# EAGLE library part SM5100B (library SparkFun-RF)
LinkSprite SM5100B GSM/GPRS Module The SM5100B is a miniature, quad-band GSM 850/EGSM 900/DCS 1800/PCS 1900 module, which can be integrated into a great number of wireless projects. You can use this module to accomplish almost anything a normal cell phone can - SMS text messages, GSM/GPRS, TCP/IP, and more! SparkFun Products GSM/GPRS Module - SM5100B (CEL-09533)
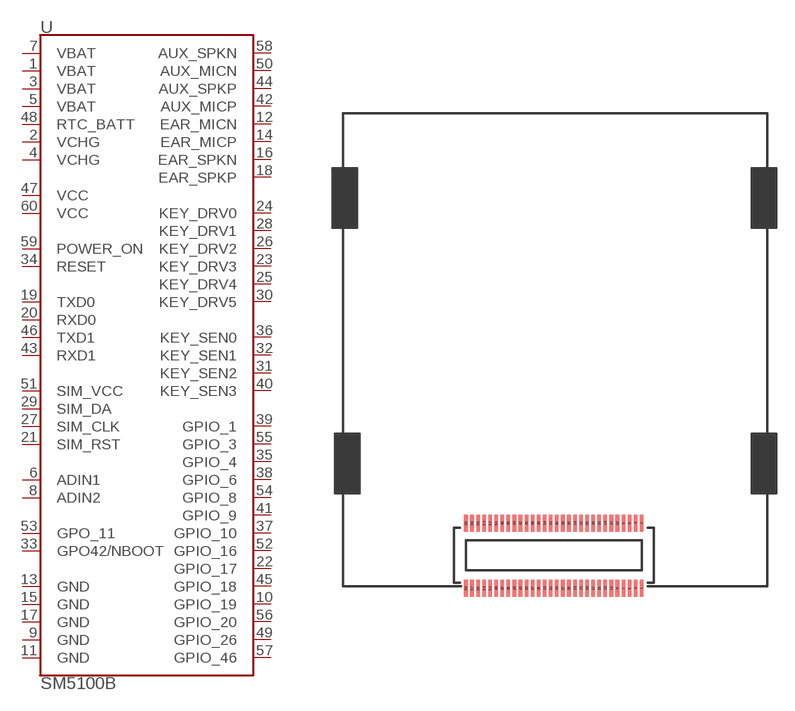
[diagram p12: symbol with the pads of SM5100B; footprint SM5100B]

Designator prefix -

## SM5100B (PROD_ID: CONN-09315)  [SM5100B]
1  VBAT
2  VCHG
3  VBAT
4  VCHG
5  VBAT
6  ADIN1
7  VBAT
8  ADIN2
9  GND
10  GPIO_19
11  GND
12  EAR_MICN
13  GND
14  EAR_MICP
15  GND
16  EAR_SPKN
17  GND
18  EAR_SPKP
19  TXD0
20  RXD0
21  SIM_RST
22  GPIO_17
23  KEY_DRV3
24  KEY_DRV0
25  KEY_DRV4
26  KEY_DRV2
27  SIM_CLK
28  KEY_DRV1
29  SIM_DA
30  KEY_DRV5
31  KEY_SEN2
32  KEY_SEN1
33  GPO42/NBOOT
34  RESET
35  GPIO_4
36  KEY_SEN0
37  GPIO_10
38  GPIO_6
39  GPIO_1
40  KEY_SEN3
41  GPIO_9
42  AUX_MICP
43  RXD1
44  AUX_SPKP
45  GPIO_18
46  TXD1
47  VCC
48  RTC_BATT
49  GPIO_26
50  AUX_MICN
51  SIM_VCC
52  GPIO_16
53  GPO_11
54  GPIO_8
55  GPIO_3
56  GPIO_20
57  GPIO_46
58  AUX_SPKN
59  POWER_ON
60  VCC

## Footprint SM5100B (pad centres in mm)
SM5100B GSM/GPRS Module - 60-pin 0.5mm-pitch board-to-board connector Mill layers define four shielding GND tabs. The SM5100B GSM/GPRS module interfaces with a board via a 60-pin board-to-board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
smd 0.3 x 1.4: 1 7.25,-2.68; 2 7.25,2.68; 3 6.75,-2.68; 4 6.75,2.68; 5 6.25,-2.68; 6 6.25,2.68; 7 5.75,-2.68; 8 5.75,2.68; 9 5.25,-2.68; 10 5.25,2.68; 11 4.75,-2.68; 12 4.75,2.68; 13 4.25,-2.68; 14 4.25,2.68; 15 3.75,-2.68; 16 3.75,2.68; 17 3.25,-2.68; 18 3.25,2.68; 19 2.75,-2.68; 20 2.75,2.68; 21 2.25,-2.68; 22 2.25,2.68; 23 1.75,-2.68; 24 1.75,2.68; 25 1.25,-2.68; 26 1.25,2.68; 27 0.75,-2.68; 28 0.75,2.68; 29 0.25,-2.68; 30 0.25,2.68; 31 -0.25,-2.68; 32 -0.25,2.68; 33 -0.75,-2.68; 34 -0.75,2.68; 35 -1.25,-2.68; 36 -1.25,2.68; 37 -1.75,-2.68; 38 -1.75,2.68; 39 -2.25,-2.68; 40 -2.25,2.68; 41 -2.75,-2.68; 42 -2.75,2.68; 43 -3.25,-2.68; 44 -3.25,2.68; 45 -3.75,-2.68; 46 -3.75,2.68; 47 -4.25,-2.68; 48 -4.25,2.68; 49 -4.75,-2.68; 50 -4.75,2.68; 51 -5.25,-2.68; 52 -5.25,2.68; 53 -5.75,-2.68; 54 -5.75,2.68; 55 -6.25,-2.68; 56 -6.25,2.68; 57 -6.75,-2.68; 58 -6.75,2.68; 59 -7.25,-2.68; 60 -7.25,2.68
